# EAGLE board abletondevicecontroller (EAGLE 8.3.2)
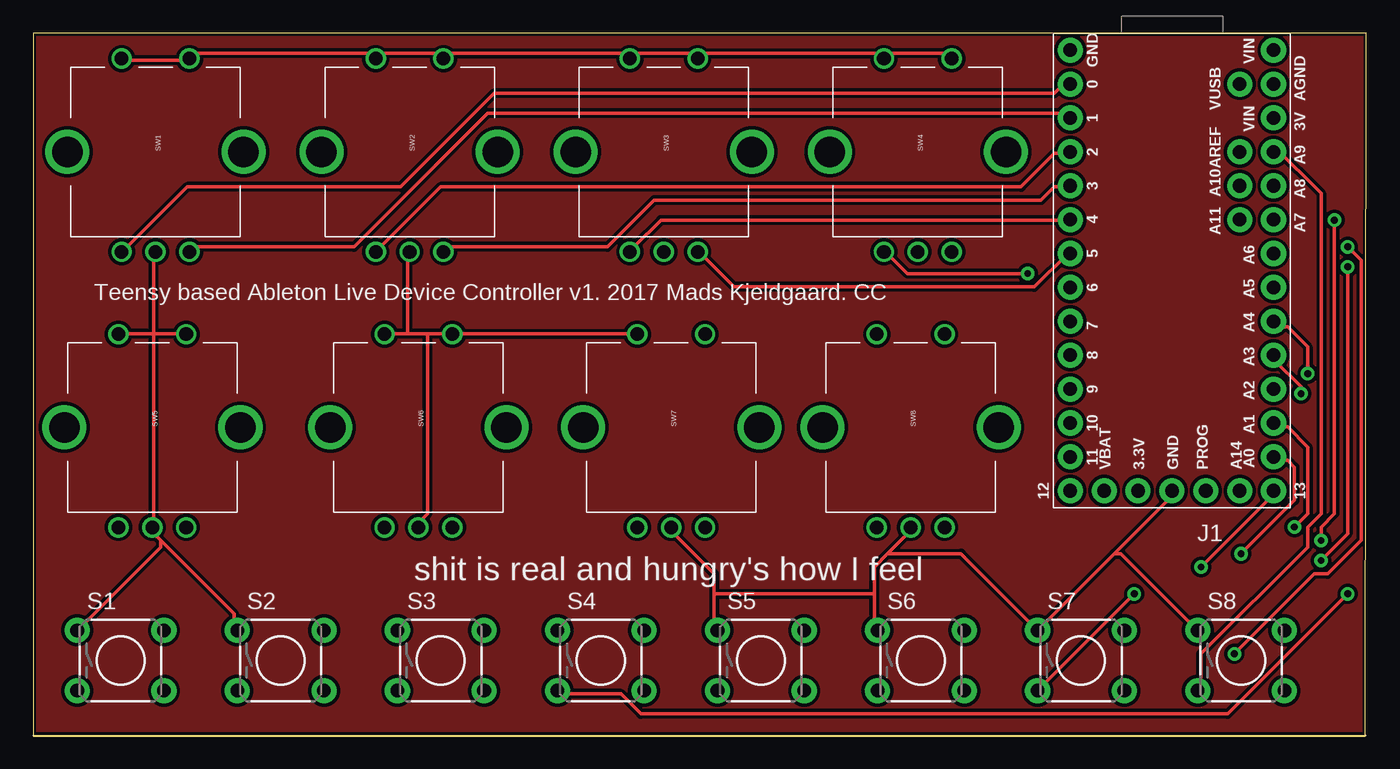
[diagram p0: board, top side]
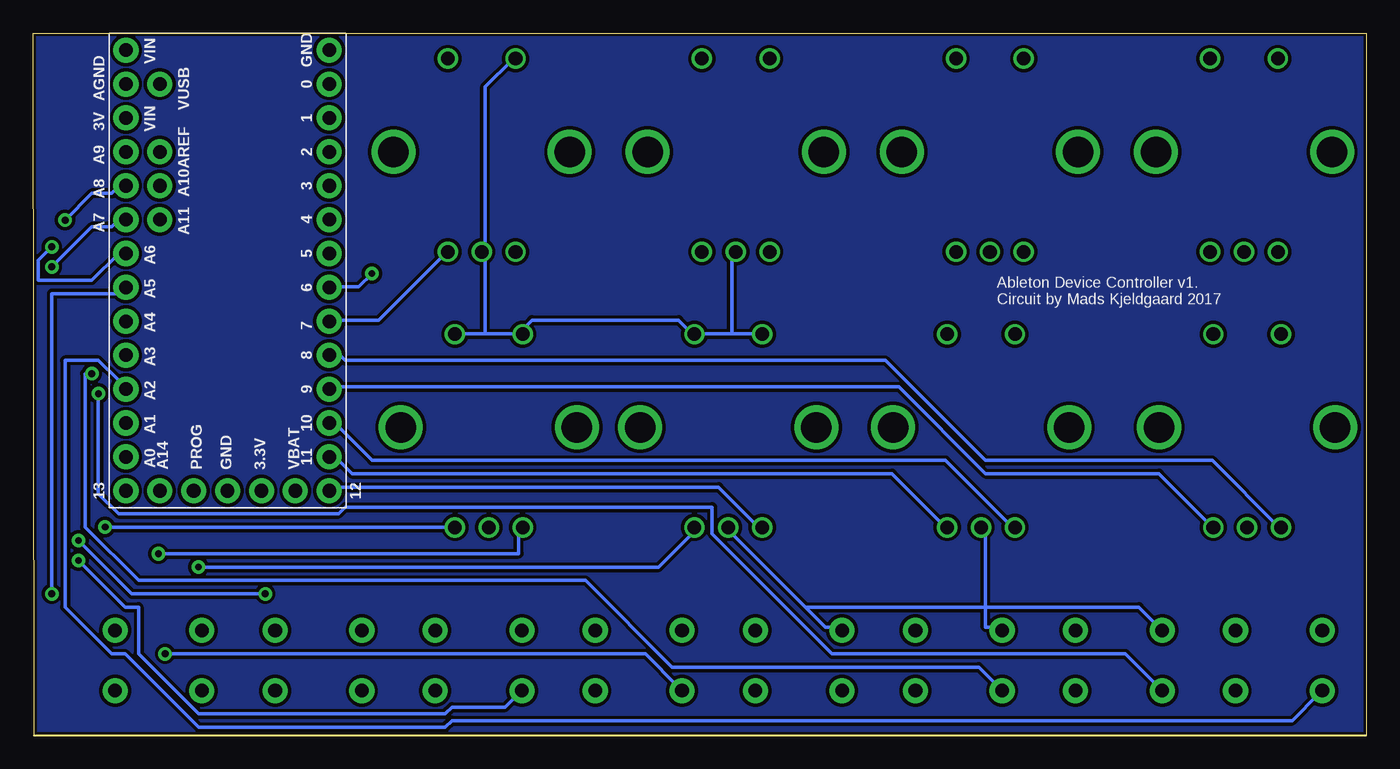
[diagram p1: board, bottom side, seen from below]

Size 99.92 x 52.63 mm. Coordinates in mm from the lower left corner, seen from the top.
Outline: 99.87,0 99.92,52.63 0,52.63 0,0 99.87,0
Copper layers (1*16): Top 0.035mm / dielectric 1.5mm / Bottom 0.035mm
Design rules "SparkFun-2-layer-STANDARD": minimum track width 10mil, minimum drill 20mil, track to track 10mil, track to pad 8mil, pad to pad 8mil, via to via 10mil, smd to smd 8mil, copper to edge 8mil, drill to drill 8mil, minimum pad ring 10mil, minimum via ring 10mil, stop-mask expansion 4mil, vias tented up to drill 25mil, thermal gap 10mil

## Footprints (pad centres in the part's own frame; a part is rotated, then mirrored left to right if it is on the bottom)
TEENSY-3.1 = drill 1.016 pad 1.88: 0 16.51,3.81; 1 16.51,6.35; 2 16.51,8.89; 3 16.51,11.43; 3.3V 11.43,34.29; 3V 1.27,6.35; 4 16.51,13.97; 5 16.51,16.51; 6 16.51,19.05; 7 16.51,21.59; 8 16.51,24.13; 9 16.51,26.67; 10 16.51,29.21; 11 16.51,31.75; 12 16.51,34.29; 13 1.27,34.29; 14 1.27,31.75; 15 1.27,29.21; 16 1.27,26.67; 17 1.27,24.13; 18 1.27,21.59; 19 1.27,19.05; 20 1.27,16.51; 21 1.27,13.97; 22 1.27,11.43; 23 1.27,8.89; A10 3.81,11.43; A11 3.81,13.97; A14/DAC 3.81,34.29; AGND 1.27,3.81; AREF 3.81,8.89; GND 8.89,34.29; GND1 16.51,1.27; PROG 6.35,34.29; VBAT 13.97,34.29; VIN 1.27,1.27; VUSB 3.81,3.81
TACTILE-PTH = drill 1.016 pad 1.88: 1 -3.251,2.261; 2 3.251,2.261; 3 -3.251,-2.261; 4 3.251,-2.261
ROTARY_ENC_PLAIN = drill 1.016: A 7.493,-2.54; B 7.493,2.54; C 7.493,0; SW+ -6.985,2.54; SW- -6.985,-2.54 | drill 2.286: P$3 0,6.604; P$4 0,-6.604

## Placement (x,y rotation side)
J1  TEENSY-3.1SILK  [TEENSY-3.1]  94.25,52.64 180 top
S1  SWITCH-MOMENTARY-2PTH  [TACTILE-PTH]  6.54,5.63 0 top
S2  SWITCH-MOMENTARY-2PTH  [TACTILE-PTH]  18.54,5.63 0 top
S3  SWITCH-MOMENTARY-2PTH  [TACTILE-PTH]  30.54,5.63 0 top
S4  SWITCH-MOMENTARY-2PTH  [TACTILE-PTH]  42.54,5.63 0 top
S5  SWITCH-MOMENTARY-2PTH  [TACTILE-PTH]  54.54,5.63 0 top
S6  SWITCH-MOMENTARY-2PTH  [TACTILE-PTH]  66.54,5.63 0 top
S7  SWITCH-MOMENTARY-2PTH  [TACTILE-PTH]  78.54,5.63 0 top
S8  SWITCH-MOMENTARY-2PTH  [TACTILE-PTH]  90.54,5.63 0 top
SW1  ROTARTY_ENCODER  [ROTARY_ENC_PLAIN]  9.16,43.75 270 top
SW2  ROTARTY_ENCODER  [ROTARY_ENC_PLAIN]  28.21,43.75 270 top
SW3  ROTARTY_ENCODER  [ROTARY_ENC_PLAIN]  47.26,43.75 270 top
SW4  ROTARTY_ENCODER  [ROTARY_ENC_PLAIN]  66.31,43.75 270 top
SW5  ROTARTY_ENCODER  [ROTARY_ENC_PLAIN]  8.92,23.1 270 top
SW6  ROTARTY_ENCODER  [ROTARY_ENC_PLAIN]  28.87,23.1 270 top
SW7  ROTARTY_ENCODER  [ROTARY_ENC_PLAIN]  47.82,23.1 270 top
SW8  ROTARTY_ENCODER  [ROTARY_ENC_PLAIN]  65.77,23.1 270 top

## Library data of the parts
J1 = SparkFun-Boards; SF_ID: DEV-12646
S1-S8 = SparkFun-Electromechanical; PROD_ID: SWCH-08441
SW1-SW8 = SparkFun-Electromechanical

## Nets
GND: J1.GND S1.1 S2.1 S3.1 S4.1 S5.1 S6.1 S7.1 S8.1 SW1.C SW1.SW+ SW1.SW- SW2.C SW2.SW+ SW2.SW- SW3.C SW3.SW+ SW3.SW- SW4.C SW4.SW+ SW4.SW- SW5.C SW5.SW+ SW5.SW- SW6.C SW6.SW+ SW6.SW- SW7.C SW7.SW+ SW7.SW- SW8.C SW8.SW+ SW8.SW-
N$1: J1.8 SW5.A
N$2: J1.9 SW5.B
N$3: J1.10 SW6.A
N$4: J1.0 SW1.A
N$5: J1.1 SW1.B
N$6: J1.2 SW2.A
N$7: J1.3 SW2.B
N$8: J1.4 SW3.A
N$9: J1.5 SW3.B
N$10: J1.6 SW4.A
N$11: J1.7 SW4.B
N$12: J1.11 SW6.B
N$13: J1.12 SW7.A
N$14: J1.13 SW7.B
N$15: J1.14 SW8.A
N$16: J1.15 SW8.B
N$17: J1.16 S1.3
N$18: J1.17 S2.3
N$19: J1.20 S5.3
N$20: J1.19 S4.3
N$21: J1.21 S6.3
N$22: J1.22 S7.3
N$23: J1.23 S8.3
N$28: J1.18 S3.3

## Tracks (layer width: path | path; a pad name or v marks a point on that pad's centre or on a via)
GND
  Top 0.254: SW4.SW+ 68.54,51.13 64.04,51.13 SW4.SW- 63.54,51.13 50.04,51.13 SW3.SW+ 49.54,51.13 45.04,51.13 SW3.SW- 44.54,51.13 31.04,51.13 SW2.SW+ 30.54,51.13 26.04,51.13 SW2.SW- 25.54,51.13 12.04,51.13 SW1.SW+ 11.54,50.63 7.04,50.63 SW1.SW- | 9.04,30.13 11.04,30.13 SW5.SW+ | 9.04,30.13 6.54,30.13 SW5.SW- | 9.04,30.13 9.04,36.13 SW1.C | 9.54,14.63 15.04,9.13 15.04,8.13 S2.1 | 9.54,14.63 9.04,15.13 SW5.C 9.04,15.63 9.04,30.13 | 9.54,14.63 9.54,14.13 3.54,8.13 S1.1 | 81.04,13.63 85.54,18.13 J1.GND | 81.04,13.63 75.54,8.13 S7.1 75.04,8.13 69.54,13.63 64.04,13.63 | 81.04,13.63 81.54,13.63 87.04,8.13 S8.1 | 64.04,13.63 63.04,12.63 63.04,10.63 | 64.04,13.63 65.54,15.13 SW8.C | 63.04,10.63 63.04,8.13 S6.1 | 29.54,30.13 31.04,30.13 SW6.SW+ 31.54,30.13 45.04,30.13 SW7.SW- | 29.54,30.13 28.04,30.13 | 28.04,30.13 26.54,30.13 SW6.SW- | 28.04,30.13 28.04,36.13 SW2.C | 51.04,10.63 51.04,12.13 48.04,15.13 SW7.C | 51.04,10.63 51.04,8.13 S5.1 | 29.54,30.13 29.54,16.63 28.54,15.63 SW6.C | 51.04,10.63 63.04,10.63
  Bottom 0.254: 47.54,30.13 50.04,30.13 SW7.SW+ 50.54,30.13 51.54,31.13 62.54,31.13 63.54,30.13 | 47.54,30.13 45.54,30.13 SW7.SW- | 47.54,30.13 47.54,36.13 SW3.C | 66.04,30.13 68.04,30.13 SW8.SW+ | 66.04,30.13 63.54,30.13 | 66.04,30.13 66.04,36.13 SW4.C 66.04,36.63 66.04,48.63 64.04,50.63 SW4.SW- | 63.54,30.13 SW8.SW- | 28.54,9.63 28.54,8.13 27.54,8.13 S3.1 | 28.54,9.63 28.54,15.13 SW6.C | 42.04,9.63 40.54,8.13 39.54,8.13 S4.1 | 42.04,9.63 47.54,15.13 SW7.C | 42.04,9.63 28.54,9.63 | 28.54,9.63 17.04,9.63 15.54,8.13 S2.1
N$1
  Bottom 0.254: SW5.A 6.54,15.63 11.54,20.63 28.54,20.63 36.04,28.13 76.54,28.13 77.04,28.63 77.54,28.63 J1.8
N$2
  Bottom 0.254: SW5.B 11.54,15.63 15.54,19.63 28.54,19.63 35.04,26.13 77.54,26.13 J1.9
N$3
  Bottom 0.254: SW6.A 26.54,15.63 31.54,20.63 74.54,20.63 77.04,23.13 77.54,23.13 J1.10
N$4
  Top 0.254: SW1.A 7.04,36.63 11.54,41.13 27.54,41.13 34.54,48.13 76.54,48.13 77.54,49.13 J1.0
N$5
  Top 0.254: SW1.B 12.04,36.63 24.04,36.63 34.04,46.63 77.54,46.63 J1.1
N$6
  Top 0.254: SW2.A 26.04,36.63 30.54,41.13 74.04,41.13 76.54,43.63 77.54,43.63 J1.2
N$7
  Top 0.254: SW2.B 31.04,36.63 43.04,36.63 46.54,40.13 75.54,40.13 76.54,41.13 77.54,41.13 J1.3
N$8
  Top 0.254: SW3.A 45.04,36.63 47.04,38.63 77.54,38.63 J1.4
N$9
  Top 0.254: SW3.B 50.04,36.13 52.54,33.63 75.04,33.63 77.54,36.13 J1.5
N$10  (via drill 0.51)
  Top 0.254: v74.54,34.63 65.54,34.63 64.04,36.13 SW4.A
  Bottom 0.254: v74.54,34.63 75.54,33.63 77.54,33.63 J1.6
N$11
  Bottom 0.254: SW4.B 69.04,36.13 74.04,31.13 77.54,31.13 J1.7
N$12
  Bottom 0.254: SW6.B 31.54,15.63 35.54,19.63 76.04,19.63 77.04,20.63 77.54,20.63 J1.11
N$13
  Bottom 0.254: SW7.A 45.54,15.63 48.54,18.63 77.54,18.63 J1.12
N$14  (via drill 0.51)
  Top 0.254: v87.54,12.63 93.04,18.13 J1.13
  Bottom 0.254: v87.54,12.63 53.04,12.63 50.54,15.13 SW7.B
N$15  (via drill 0.51)
  Top 0.254: v90.54,13.63 94.54,17.63 94.54,20.13 94.04,20.63 93.04,20.63 J1.14
  Bottom 0.254: v90.54,13.63 63.54,13.63 63.54,15.13 SW8.A
N$16  (via drill 0.51)
  Top 0.254: v94.54,15.63 95.54,16.63 95.54,21.63 94.04,23.13 93.04,23.13 J1.15
  Bottom 0.254: v94.54,15.63 68.54,15.63 SW8.B
N$17
  Bottom 0.254: S1.3 3.54,3.13 5.54,1.13 68.54,1.13 69.04,0.63 87.54,0.63 93.04,6.13 94.04,6.13 97.54,9.63 97.54,28.13 95.04,28.13 93.54,26.63 93.54,26.13 93.04,26.13 J1.16
N$18  (via drill 0.51)
  Top 0.254: v95.04,25.63 95.04,26.13 93.04,28.13 J1.17
  Bottom 0.254: v95.04,25.63 95.04,18.13 93.54,16.63 77.04,16.63 76.54,17.13 49.04,17.13 49.04,15.13 40.04,6.13 18.04,6.13 15.54,3.63 S2.3
N$19  (via drill 0.51)
  Top 0.254: v90.04,6.13 96.04,12.13 97.04,12.13 99.54,14.63 99.54,35.63 v98.54,36.63
  Bottom 0.254: v90.04,6.13 54.04,6.13 51.54,3.63 S5.3 | v98.54,36.63 99.54,35.63 99.54,34.13 95.54,34.13 93.54,36.13 J1.20
N$20  (via drill 0.51)
  Top 0.254: v98.54,10.63 89.54,1.63 45.54,1.63 44.04,3.13 39.54,3.13 S4.3
  Bottom 0.254: v98.54,10.63 98.54,33.13 93.04,33.13 J1.19
N$21  (via drill 0.51)
  Top 0.254: v96.54,13.13 98.54,15.13 v98.54,35.13
  Bottom 0.254: v96.54,13.13 93.04,9.63 92.04,9.63 92.04,6.13 87.54,1.63 69.04,1.63 68.54,2.13 64.54,2.13 63.54,3.13 S6.3 | v98.54,35.13 95.54,38.13 94.04,38.13 93.54,38.63 93.04,38.63 J1.21
N$22  (via drill 0.51)
  Top 0.254: v82.54,10.63 75.54,3.63 S7.3 | v96.54,14.63 96.54,15.63 97.54,16.63 v97.54,38.63
  Bottom 0.254: v82.54,10.63 92.54,10.63 v96.54,14.63 | v97.54,38.63 95.54,40.63 94.04,40.63 93.54,41.13 93.04,41.13 J1.22
N$23
  Top 0.254: S8.3 87.54,3.63 87.54,6.13 95.54,14.13 95.54,15.63 96.54,16.63 96.54,40.63 93.04,44.13 J1.23
N$25
  pour Top: 0,52.64 0,0 99.87,0 99.87,52.64
N$26
  pour Bottom: 0,52.64 0,0 99.87,0 99.87,52.64
N$28  (via drill 0.51)
  Top 0.254: v95.54,27.13 95.54,29.13 94.04,30.63 93.04,30.63 J1.18
  Bottom 0.254: v95.54,27.13 96.04,27.13 96.04,15.63 92.04,11.63 58.54,11.63 52.04,5.13 29.04,5.13 27.54,3.63 S3.3

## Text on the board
bPlace: Ableton Device Controller v1. / Circuit by Mads Kjeldgaard 2017
tNames: Teensy based Ableton Live Device Controller v1. 2017 Mads Kjeldgaard. CC | shit is real and hungry's how I feel

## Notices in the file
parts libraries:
SparkFun-Boards: Licensing: Creative Commons ShareAlike 4.0 International - https://creativecommons.org/licenses/by-sa/4.0
